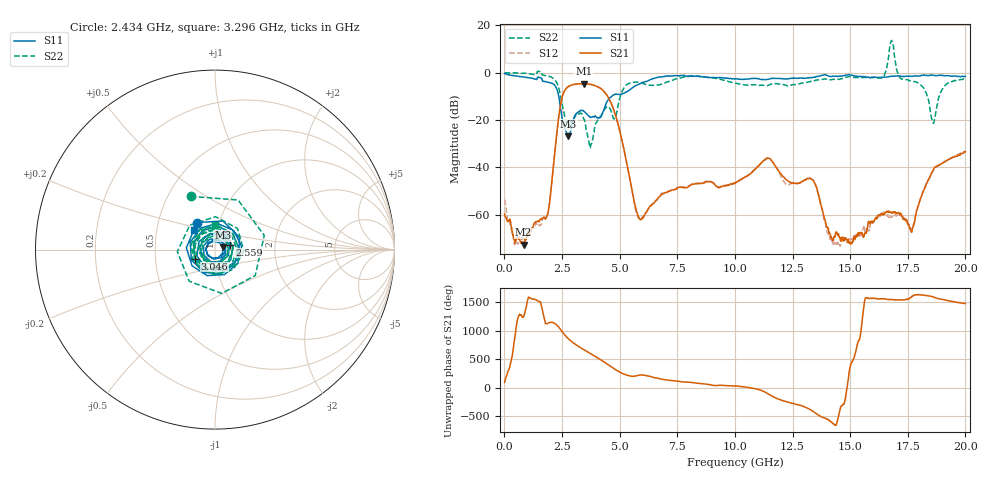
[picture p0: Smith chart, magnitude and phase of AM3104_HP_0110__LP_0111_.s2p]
!Created with skrf (http://scikit-rf.org).
# Hz S RI R 50.0
!freq ReS11 ImS11 ReS21 ImS21 ReS12 ImS12 ReS22 ImS22
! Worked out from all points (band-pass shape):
!   1601 points, 10 MHz to 20 GHz, reference 50 ohm
!   highest |S21| = -4.65 dB at 3.446 GHz (marker M1); lowest = -72.7 dB at 834.6 MHz (marker M2)
!   |S21| within 3 dB of the highest: 2.611 GHz to 4.296 GHz (1.685 GHz wide, 48.8 % of centre)
!   lowest |S11| = -26.8 dB at 2.771 GHz (marker M3), VSWR 1.10, Z = 54.6 + j1.42 ohm
!   |S11| at or under -10 dB: 2.36 GHz to 4.654 GHz (2.294 GHz wide, 65.4 % of centre)
!   |S22| runs from -31.8 to 13.6 dB; largest |S21 - S12| = 0.036
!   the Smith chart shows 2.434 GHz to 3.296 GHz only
!   S11 on the Smith chart (normalised r, x): 2.434 GHz: 0.79, +0.25; 2.559 GHz: 1.17, +0.07; 3.046 GHz: 0.80, -0.08; 3.296 GHz: 0.77, +0.17
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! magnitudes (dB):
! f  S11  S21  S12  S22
! 10 MHz  -0.3  -59.8  -53.6  0.0
! 834.6 MHz  -1.8  -72.7  -69.7  -0.2
! 1.872 GHz  -4.0  -60.0  -59.9  -1.4
! 2.434 GHz  -14.9  -13.7  -13.8  -9.7
! 2.559 GHz  -21.3  -8.7  -8.8  -15.9
! 2.771 GHz  -26.8  -5.9  -5.9  -22.6
! 3.046 GHz  -18.2  -5.0  -4.9  -18.7
! 3.296 GHz  -15.9  -4.7  -4.8  -17.1
! 3.346 GHz  -16.0  -4.7  -4.8  -17.2
! 3.446 GHz  -16.3  -4.6  -4.7  -19.6
! 3.733 GHz  -18.9  -4.9  -5.0  -31.4
! 4.683 GHz  -9.8  -14.0  -14.2  -18.0
! 5.807 GHz  -5.0  -60.6  -61.5  -4.0
! 6.682 GHz  -1.9  -52.8  -52.8  -5.2
! 10.01 GHz  -2.7  -46.8  -46.8  -4.4
! 11.43 GHz  -2.8  -36.0  -36.3  -5.4
! 13.34 GHz  -2.1  -45.1  -45.2  -3.7
! 14.33 GHz  -1.6  -69.2  -72.3  -2.8
! 16.68 GHz  -1.6  -58.9  -61.2  7.2
! 17.68 GHz  -1.6  -67.4  -65.9  -3.7
! 18.6 GHz  -1.1  -41.3  -41.5  -21.3
! 20 GHz  -1.5  -33.4  -33.2  -2.5
